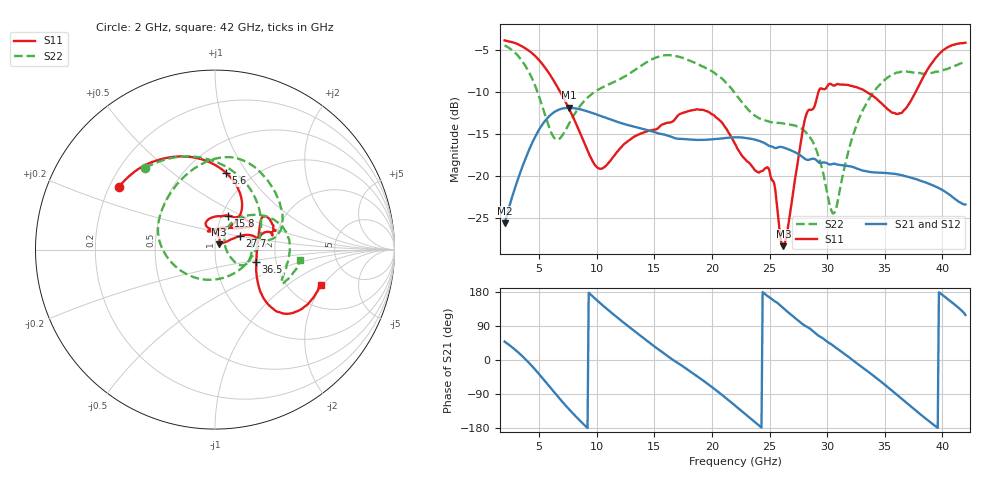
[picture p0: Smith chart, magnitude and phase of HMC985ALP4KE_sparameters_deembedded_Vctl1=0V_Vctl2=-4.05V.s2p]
!s2p File: Measurements: S11, S21, S12, S22
# GHz S dB R 50.0
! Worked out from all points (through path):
!   401 points, 2 GHz to 42 GHz, reference 50 ohm
!   highest |S21| = -11.90 dB at 7.6 GHz (marker M1); lowest = -25.7 dB at 2 GHz (marker M2)
!   lowest |S11| = -28.4 dB at 26.2 GHz (marker M3), VSWR 1.08, Z = 52.3 + j3.17 ohm
!   |S11| at or under -10 dB: 6.822 GHz to 29.25 GHz (22.43 GHz wide, 124 % of centre); 33.42 GHz to 37.69 GHz (4.271 GHz wide, 12 % of centre)
!   |S22| runs from -24.5 to -4.5 dB; largest |S21 - S12| = 0.00023
!   S11 on the Smith chart (normalised r, x): 2 GHz: 0.24, +0.28; 5.6 GHz: 0.76, +0.80; 15.8 GHz: 1.07, +0.42; 27.7 GHz: 1.30, +0.20; 36.5 GHz: 1.57, -0.23; 42 GHz: 2.95, -1.89
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2  -3.88 147.0  -25.67 48.6  -25.68 48.6  -4.47 130.5
3.6  -4.66 120.3  -18.70 8.3  -18.70 8.3  -6.48 84.9
4.6  -5.66 101.5  -15.49 -23.5  -15.49 -23.5  -9.10 47.8
5.6  -7.28 81.9  -13.30 -59.2  -13.30 -59.2  -13.11 -3.8
6.5  -9.21 66.5  -12.25 -92.1  -12.26 -92.1  -15.68 -69.4
7.6  -12.03 54.8  -11.90 -130.3  -11.91 -130.3  -13.77 -136.2
8.7  -15.38 55.0  -12.13 -164.9  -12.13 -164.9  -11.42 -170.5
10.4  -19.15 89.6  -12.90 147.3  -12.90 147.3  -9.53 162.1
15.4  -14.22 75.7  -14.97 27.1  -14.97 27.1  -5.79 86.6
15.8  -13.82 68.7  -15.07 18.2  -15.07 18.2  -5.66 81.5
19.3  -12.17 33.6  -15.71 -55.6  -15.71 -55.6  -7.03 35.8
22  -16.19 51.2  -15.41 -120.2  -15.42 -120.2  -10.16 10.1
24.9  -19.04 104.6  -16.38 167.1  -16.39 167.1  -13.51 13.2
26.2  -28.37 52.4  -16.62 136.7  -16.63 136.7  -13.77 -3.1
27.7  -16.11 28.6  -17.58 98.6  -17.58 98.6  -14.30 -24.0
28.7  -12.11 12.6  -17.97 78.1  -17.98 78.0  -15.81 -32.0
30.6  -9.26 19.5  -18.55 36.1  -18.56 36.1  -24.43 20.1
32.8  -9.59 33.9  -19.24 -13.8  -19.24 -13.8  -13.07 52.5
35.4  -12.22 11.7  -19.69 -75.1  -19.69 -75.1  -8.17 20.6
36.5  -12.47 -16.7  -19.93 -103.0  -19.93 -103.1  -7.59 6.6
39.5  -5.86 -43.7  -21.33 -176.8  -21.32 -176.8  -7.59 -26.2
42  -4.15 -18.5  -23.41 118.8  -23.41 118.7  -6.41 -6.8
